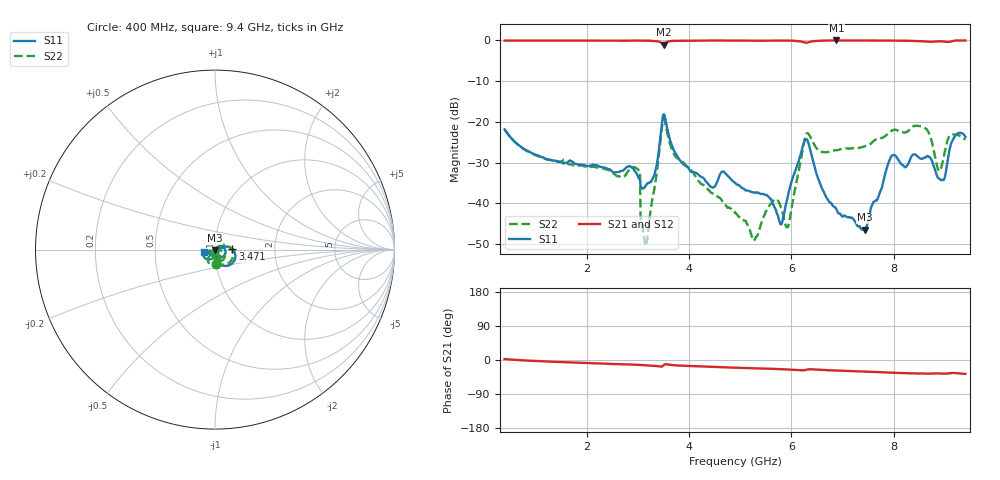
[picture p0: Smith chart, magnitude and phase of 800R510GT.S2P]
!  American Technical Ceramics  Date:  6/19/09
!  One Norden Lane
!  Huntington Station,  NY.  11746-2102
!  Tel:  (631) 622-4700  Fax:  (631) 622-4748
!  Part Number  800R510GT
!  Description: Ultra-low ESR, NPO  Mounting Orientation: Vertical
!  Application: High RF power Filters, Combiners, Matching networks,
!  Antenna, DC block, Bypass and Couplers
# GHZ S DB R 50
! Freq  |S11|  S11 Ph  |S21|  S21 Ph  |S12|  S12 Ph  |S22|  S22 Ph
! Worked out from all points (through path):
!   801 points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, 400 MHz to 9.4 GHz, reference 50 ohm
!   highest |S21| = 0.00 dB at 6.88 GHz (marker M1); lowest = -1.0 dB at 3.505 GHz (marker M2)
!   group delay of S21, straight-line fit = 11.7 ps
!   lowest |S11| = -46.5 dB at 7.431 GHz (marker M3), VSWR 1.01, Z = 49.9 - j0.451 ohm
!   |S11| at or under -10 dB: start of sweep to end of sweep
!   |S22| runs from -50.5 to -19.2 dB; largest |S21 - S12| = 0.0051
!   S11 on the Smith chart (normalised r, x): 400 MHz: 1.00, -0.16; 3.471 GHz: 1.21, +0.01; 9.4 GHz: 0.88, -0.03
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0.4  -21.82 -86.5  -0.03 2.7  -0.06 2.7  -21.81 -86.8
1.908  -30.49 -84.3  -0.02 -7.4  -0.04 -7.3  -30.70 -108.0
2.999  -33.18 -65.8  -0.01 -12.8  -0.03 -12.7  -31.58 -140.3
3.1  -36.39 -47.2  -0.03 -13.5  -0.05 -13.4  -46.48 -169.7
3.156  -35.60 -33.9  -0.05 -13.9  -0.07 -13.8  -50.49 151.0
3.404  -27.86 17.7  -0.23 -16.5  -0.25 -16.4  -29.05 40.4
3.471  -20.32 2.2  -0.77 -17.3  -0.79 -17.2  -21.38 7.6
3.505  -18.11 -28.2  -1.05 -13.8  -1.07 -13.7  -19.19 -28.6
4.034  -32.20 -73.7  -0.06 -15.9  -0.08 -15.8  -31.59 -132.7
4.9  -34.94 -49.7  -0.04 -20.3  -0.05 -20.2  -42.13 -147.2
5.283  -37.35 -31.4  -0.06 -22.0  -0.06 -21.9  -48.92 -107.0
5.789  -45.13 0.9  -0.03 -24.1  -0.04 -23.9  -40.65 -95.3
5.924  -38.69 48.3  -0.03 -25.0  -0.03 -24.8  -45.76 -55.4
6.261  -24.59 -7.5  -0.50 -26.8  -0.50 -26.6  -24.18 -28.1
6.408  -28.77 -76.0  -0.21 -24.6  -0.21 -24.4  -24.57 -83.8
6.88  -41.43 -114.8  0.00 -27.8  -0.01 -27.6  -26.94 -88.8
7.431  -46.48 -107.6  -0.01 -30.4  -0.01 -30.2  -26.02 -84.1
7.904  -29.83 -96.7  -0.01 -33.3  -0.01 -33.1  -22.71 -80.5
8.59  -28.80 -151.6  -0.22 -35.9  -0.20 -35.7  -21.32 -109.8
8.95  -34.24 -133.4  -0.23 -36.0  -0.21 -35.8  -30.13 -61.6
9.164  -24.18 -118.0  -0.11 -34.2  -0.09 -33.9  -23.05 -70.6
9.4  -23.67 -167.2  -0.01 -36.6  -0.01 -36.3  -24.37 -77.2
